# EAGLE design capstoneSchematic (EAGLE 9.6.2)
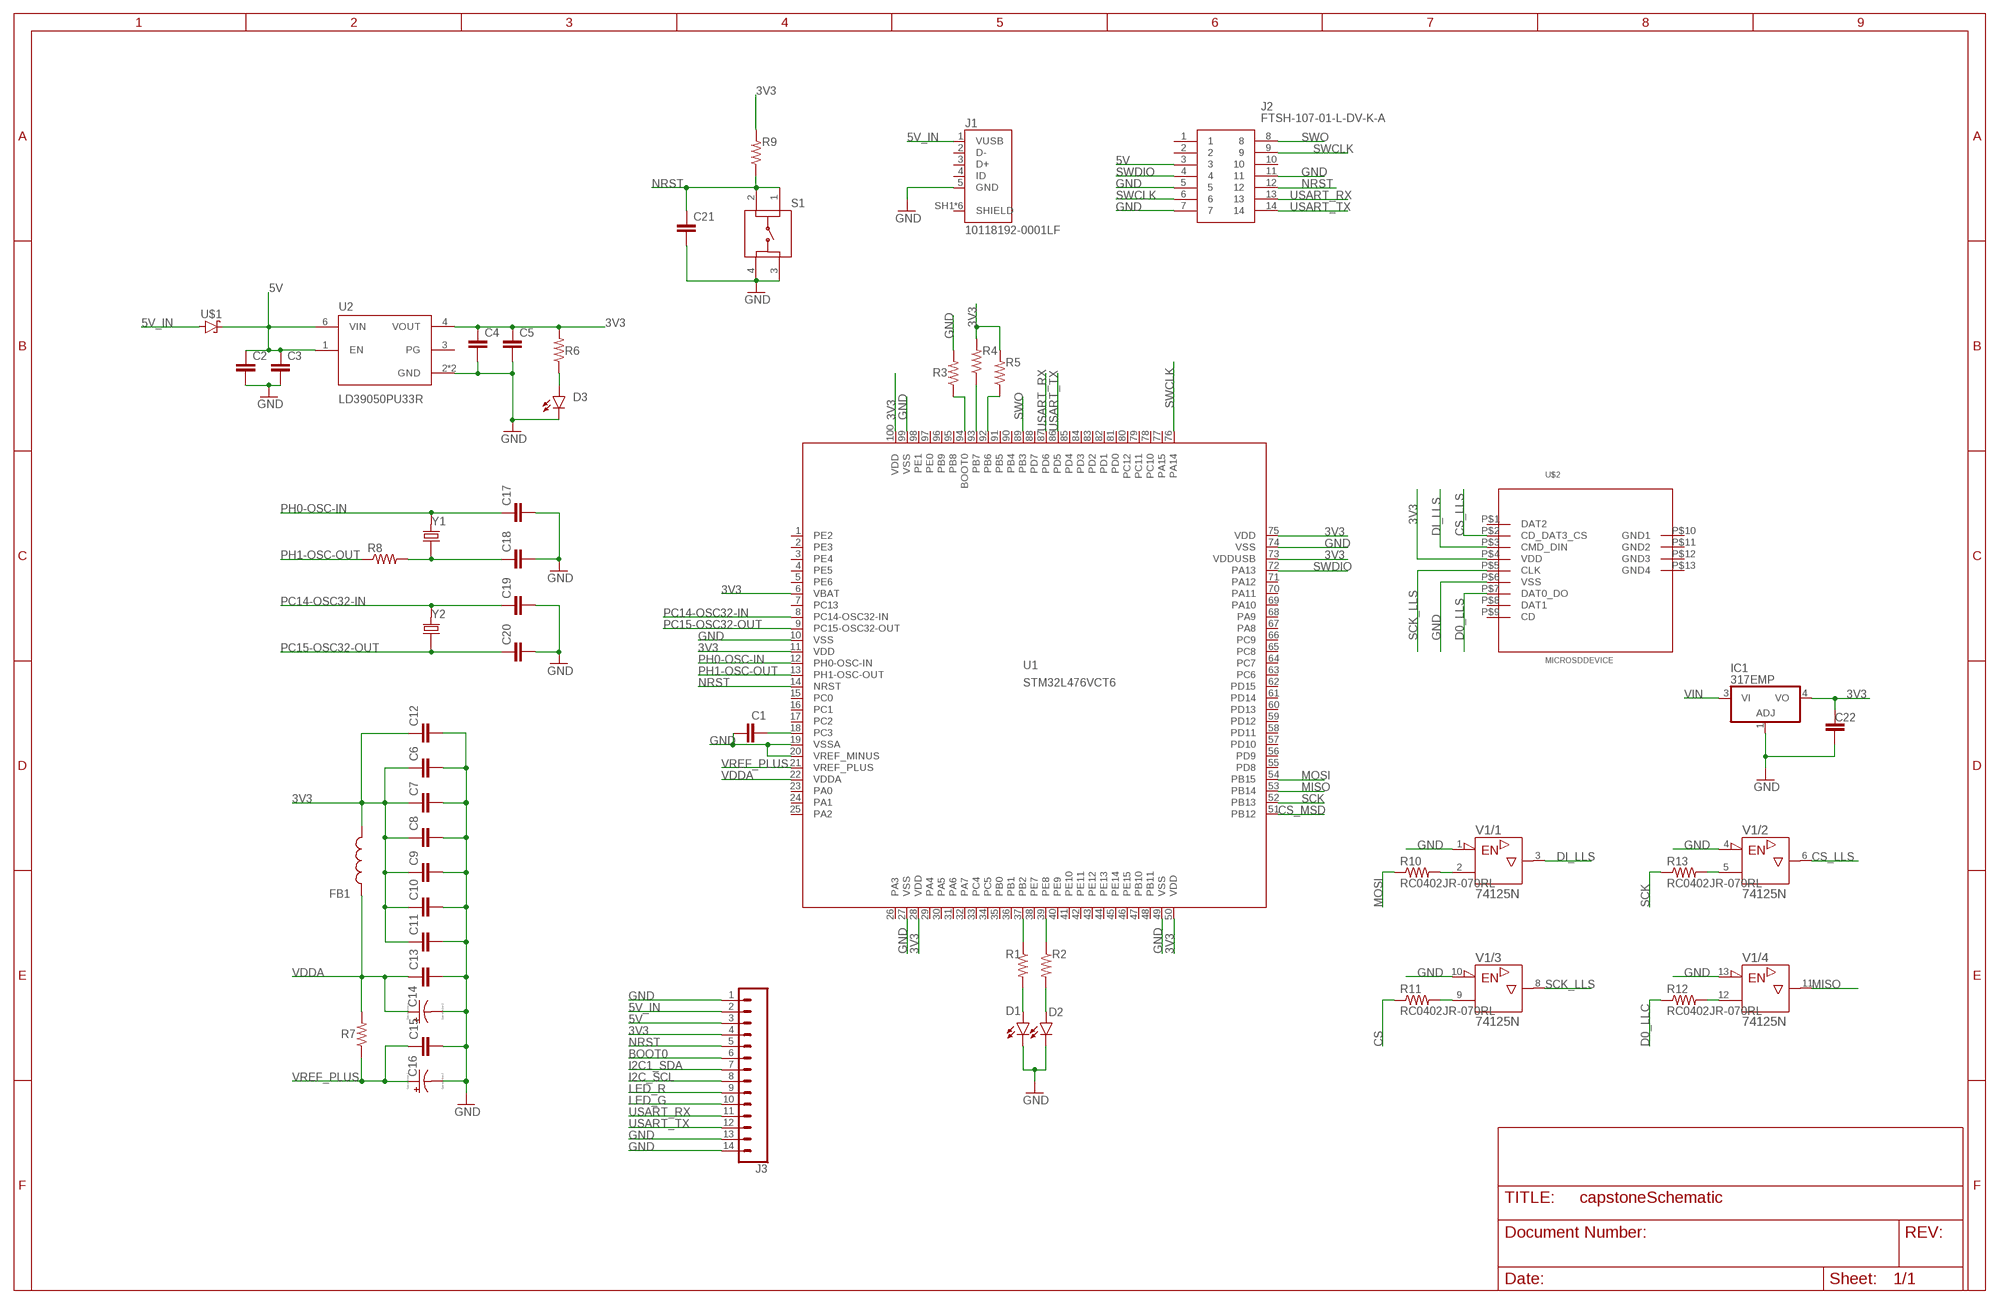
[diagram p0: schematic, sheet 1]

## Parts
C1  CC0603KRX5R7BB105  [CAPC1608X90]
C2  CC0603KRX5R7BB105  [CAPC1608X90]
C3  CC0402KRX7R7BB104  [CAPC1005X55N]
C4  CC0603KRX5R7BB105  [CAPC1608X90]
C5  CC0402KRX7R7BB104  [CAPC1005X55N]
C6  CC0402KRX7R7BB104  [CAPC1005X55N]
C7  CC0402KRX7R7BB104  [CAPC1005X55N]
C8  CC0402KRX7R7BB104  [CAPC1005X55N]
C9  CC0402KRX7R7BB104  [CAPC1005X55N]
C10  CC0402KRX7R7BB104  [CAPC1005X55N]
C11  CC0402KRX7R7BB104  [CAPC1005X55N]
C12  CC0603KRX5R7BB105  [CAPC1608X90]
C13  CC0402KRX7R7BB104  [CAPC1005X55N]
C14  TAJA105K016RNJ  [CAPPM3216X180N]
C15  CC0402KRX7R7BB104  [CAPC1005X55N]
C16  TAJA105K016RNJ  [CAPPM3216X180N]
C17  CC0402JRNPO9BN200  [CAPC1005X55N]
C18  CC0402JRNPO9BN200  [CAPC1005X55N]
C19  CC0402CRNPO9BN4R7  [CAPC1005X55N]
C20  CC0402CRNPO9BN4R7  [CAPC1005X55N]
C21  CC0402KRX7R7BB104  [CAPC1005X55N]
C22  C  (no package)
D1  SML-P12MTT86  [LED_SML-P11UTT86R]
D2  SML-P12MTT86  [LED_SML-P11UTT86R]
D3  SML-P12MTT86  [LED_SML-P11UTT86R]
FB1  BK1608HS601-T  [BEADC1608X95N]
IC1  317EMP  [SOT223]
J1  10118192-0001LF  [AMPHENOL_10118192-0001LF]
J2  FTSH-107-01-L-DV-K-A  [FTSH10701LDVKA]
J3  CONN_14  [1X14]
R1  RC0402FR-071KL  [RESC1005X40N]
R2  RC0402FR-071KL  [RESC1005X40N]
R3  RC0402FR-071KL  [RESC1005X40N]
R4  RC0402FR-071KL  [RESC1005X40N]
R5  RC0402FR-071KL  [RESC1005X40N]
R6  RC0402FR-071KL  [RESC1005X40N]
R7  RC0402FR-071KL  [RESC1005X40N]
R8  RC0402FR-072KL  [RESC1005X40N]
R9  RC0402FR-0710KL  [RESC1005X40N]
R10  RC0402JR-070RL  [RESC1005X40]
R11  RC0402JR-070RL  [RESC1005X40]
R12  RC0402JR-070RL  [RESC1005X40]
R13  RC0402JR-070RL  [RESC1005X40]
S1  LL3301FF065QJ  [LL3301FF065QJ]
U1  STM32L476VCT6  [LQFP100_14X14]
U2  LD39050PU33R  [SON95P300X300X100-7N]
U$1  STPS1L30A  [DIOM5226X223N]
U$2  MICROSDDEVICE  [MICROSD]
V1  74125N  [DIL14]
Y1  ABLS-8.000MHZ-B2-T  [XTAL_ABLS-8.000MHZ-B2-T]
Y2  ECS-.327-12.5-12QS-TR  [XTAL_ECS-.327-12.5-12QS-TR]

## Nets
3V3: C4.1 C5.1 C6.1 C7.1 C8.1 C9.1 C10.1 C11.1 C12.1 C22.1 FB1.2 IC1.4(VO) J3.4 R4.2 R5.2 R6.2 R9.2 U1.6(VBAT) U1.11(VDD) U1.28(VDD) U1.50(VDD) U1.73(VDDUSB) U1.75(VDD) U1.100(VDD) U2.4(VOUT) U$2.P$4(VDD)
5V: C2.1 C3.1 J2.3 J3.3 U2.1(EN) U2.6(VIN) U$1.1(C)
5V_IN: J1.1(VUSB) J3.2 U$1.2(A)
BOOT0: J3.6
CS: R11.1
CS_LLS: U$2.P$2(CD_DAT3_CS) V1.6(/2:Y)
CS_MSD: U1.51(PB12)
D0_LLC: R12.1
D0_LLS: U$2.P$7(DAT0_DO)
DI_LLS: U$2.P$3(CMD_DIN) V1.3(/1:Y)
GND: C1.1 C2.2 C3.2 C4.2 C5.2 C6.2 C7.2 C8.2 C9.2 C10.2 C11.2 C12.2 C13.2 C14.C(-) C15.2 C16.C(-) C17.2 C18.2 C19.2 C20.2 C21.2 C22.2 D1.C D2.C D3.C IC1.1(ADJ) J1.5(GND) J2.5 J2.7 J2.11 J3.1 J3.13 J3.14 R3.2 S1.3 S1.4 U1.10(VSS) U1.19(VSSA) U1.20(VREF_MINUS) U1.27(VSS) U1.49(VSS) U1.74(VSS) U1.99(VSS) U2.2(GND) U2.7(GND) U$2.P$6(VSS) V1.1(/1:!G) V1.4(/2:!G) V1.10(/3:!G) V1.13(/4:!G)
I2C1_SDA: J3.7
I2C_SCL: J3.8
LED_G: J3.10
LED_R: J3.9
MISO: U1.53(PB14) V1.11(/4:Y)
MOSI: R10.1 U1.54(PB15)
N$1: R2.1 U1.39(PE8)
N$2: R1.1 U1.37(PB2)
N$3: D1.A R1.2
N$4: D2.A R2.2
N$5: R3.1 U1.94(BOOT0)
N$6: R4.1 U1.93(PB7)
N$7: R5.1 U1.92(PB6)
N$8: D3.A R6.1
N$10: C1.2 U1.18(PC3)
N$12: C18.1 R8.2 Y1.1
N$13: R10.2 V1.2(/1:A)
N$15: R11.2 V1.9(/3:A)
N$17: R13.2 V1.5(/2:A)
N$21: R12.2 V1.12(/4:A)
NRST: C21.1 J2.12 J3.5 R9.1 S1.1 S1.2 U1.14(NRST)
PC14-OSC32-IN: C19.1 U1.8(PC14-OSC32-IN) Y2.2
PC15-OSC32-OUT: C20.1 U1.9(PC15-OSC32-OUT) Y2.1
PH0-OSC-IN: C17.1 U1.12(PH0-OSC-IN) Y1.2
PH1-OSC-OUT: R8.1 U1.13(PH1-OSC-OUT)
SCK: R13.1 U1.52(PB13)
SCK_LLS: U$2.P$5(CLK) V1.8(/3:Y)
SWCLK: J2.6 J2.9 U1.76(PA14)
SWDIO: J2.4 U1.72(PA13)
SWO: J2.8 U1.89(PB3)
USART_RX: J2.13 J3.11 U1.87(PD6)
USART_TX: J2.14 J3.12 U1.86(PD5)
VDDA: C13.1 C14.A(+) FB1.1 R7.2 U1.22(VDDA)
VIN: IC1.3(VI)
VREF_PLUS: C15.1 C16.A(+) R7.1 U1.21(VREF_PLUS)
Unconnected: J1.2(D-) J1.3(D+) J1.4(ID) J1.SH1(SHIELD) J1.SH2(SHIELD) J1.SH3(SHIELD) J1.SH4(SHIELD) J1.SH5(SHIELD) J1.SH6(SHIELD) J2.1 J2.2 J2.10 U1.1(PE2) U1.2(PE3) U1.3(PE4) U1.4(PE5) U1.5(PE6) U1.7(PC13) U1.15(PC0) U1.16(PC1) U1.17(PC2) U1.23(PA0) U1.24(PA1) U1.25(PA2) U1.26(PA3) U1.29(PA4) U1.30(PA5) U1.31(PA6) U1.32(PA7) U1.33(PC4) U1.34(PC5) U1.35(PB0) U1.36(PB1) U1.38(PE7) U1.40(PE9) U1.41(PE10) U1.42(PE11) U1.43(PE12) U1.44(PE13) U1.45(PE14) U1.46(PE15) U1.47(PB10) U1.48(PB11) U1.55(PD8) U1.56(PD9) U1.57(PD10) U1.58(PD11) U1.59(PD12) U1.60(PD13) U1.61(PD14) U1.62(PD15) U1.63(PC6) U1.64(PC7) U1.65(PC8) U1.66(PC9) U1.67(PA8) U1.68(PA9) U1.69(PA10) U1.70(PA11) U1.71(PA12) U1.77(PA15) U1.78(PC10) U1.79(PC11) U1.80(PC12) U1.81(PD0) U1.82(PD1) U1.83(PD2) U1.84(PD3) U1.85(PD4) U1.88(PD7) U1.90(PB4) U1.91(PB5) U1.95(PB8) U1.96(PB9) U1.97(PE0) U1.98(PE1) U2.3(PG) U$2.P$1(DAT2) U$2.P$8(DAT1) U$2.P$9(CD) U$2.P$10(GND1) U$2.P$11(GND2) U$2.P$12(GND3) U$2.P$13(GND4)

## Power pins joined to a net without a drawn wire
+UB: V1.14(/+UB:+UB)
-UB: V1.7(/-UB:-UB)

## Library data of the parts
C1 C2 C4 C12 = ce-capstone:CC0603KRX5R7BB105: CAPACITOR CERAMIC, 1µF, 10V, X5R, 0603; Dielectric Characteristic:X5R; Capacitance:1µF; Capacitance Tolerance:± 10%; Voltage Rating:16V; Temperature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; DESCRIPTION: 1µF ±10% 16V Ceramic Capacitor X5R 0603 _1608 Metric_; DIGI-KEY_PART_NUMBER: 311-1444-1-ND; DIGI-KEY_PURCHASE_URL: https://www.digikey.com/product-detail/en/yageo/CC0603KRX5R7BB105/311-1444-1-ND/2833750?utm_source=snapeda&utm_medium=aggregator&utm_campaign=symbol; MF: Yageo; MP: CC0603KRX5R7BB105; PACKAGE: 0603 Yageo
C3 C5-C11 C13 C15 C21 = ce-capstone:CC0402KRX7R7BB104: .1UF 16V 10% 0402; DESCRIPTION: 0.1µF ±10% 16V Ceramic Capacitor X7R 0402 _1005 Metric_; DIGI-KEY_PART_NUMBER: 311-1338-1-ND; DIGI-KEY_PURCHASE_URL: https://www.digikey.com/product-detail/en/yageo/CC0402KRX7R7BB104/311-1338-1-ND/2103122?utm_source=snapeda&utm_medium=aggregator&utm_campaign=symbol; MF: Yageo; MP: CC0402KRX7R7BB104; PACKAGE: 0402 Yageo
C14 C16 = ce-capstone:TAJA105K016RNJ: Capacitor tantalum TAJ 1206 1uF 16V AVX 1uF SMD Solid MnO2 Tantalum Electrolytic Capacitor, 16 V dc +/-10%, TAJ Series; ALLIED_NUMBER: 70474975; ALLIED_PRICE-STOCK: https://www.alliedelec.com/avx-taja105k016r/70474975/; DESCRIPTION: Capacitor tantalum TAJ 1206 1uF 16V AVX 1uF SMD Solid MnO2 Tantalum Electrolytic Capacitor, 16 V dc +/-10%, TAJ Series; HEIGHT: 1.8mm; MANUFACTURER_NAME: AVX; MANUFACTURER_PART_NUMBER: TAJA105K016RNJ; MOUSER_PART_NUMBER: 581-TAJA105K016RNJ; MOUSER_PRICE-STOCK: https://www.mouser.com/Search/Refine.aspx?Keyword=581-TAJA105K016R; RS_PART_NUMBER: 6992804P; RS_PRICE-STOCK: http://uk.rs-online.com/web/p/products/6992804P
C17 C18 = ce-capstone:CC0402JRNPO9BN200: CAPACITOR CERAMIC 20PF 50V, C0G, 0402; Dielectric Characteristic:C0G / NP0; Capacitance:20pF; Capacitance Tolerance:± 5%; Voltage Rating:50V; Capacitor Case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; DESCRIPTION: 20pF ±5% 50V Ceramic Capacitor C0G, NP0 0402 _1005 Metric_; DIGI-KEY_PART_NUMBER: 311-1417-1-ND; DIGI-KEY_PURCHASE_URL: https://www.digikey.com/product-detail/en/yageo/CC0402JRNPO9BN200/311-1417-1-ND/2833723?utm_source=snapeda&utm_medium=aggregator&utm_campaign=symbol; MF: Yageo; MP: CC0402JRNPO9BN200; PACKAGE: 0402 Yageo
C19 C20 = ce-capstone:CC0402CRNPO9BN4R7: 0402 4.7 pF 50 V ±0.25 pF Tolerance NP0 SMT Multilayer Ceramic Capacitor; DESCRIPTION: 4.7pF ±0.25pF 50V Ceramic Capacitor C0G, NP0 0402 _1005 Metric_; DIGI-KEY_PART_NUMBER: 311-1367-1-ND; DIGI-KEY_PURCHASE_URL: https://www.digikey.com/product-detail/en/yageo/CC0402CRNPO9BN4R7/311-1367-1-ND/2103151?utm_source=snapeda&utm_medium=aggregator&utm_campaign=symbol; MF: Yageo; MP: CC0402CRNPO9BN4R7; PACKAGE: 0402 Yageo
C22 = ngspice-simulation:C: CAPACITOR
D1-D3 = ce-capstone:SML-P12MTT86: SML-P1 Series Red 0402 Clear 60 mcd 2 V Surface Mount PICOLED LED; AVAILABILITY: Unavailable; DESCRIPTION: Green 572nm LED Indication - Discrete 2V 0402 _1006 Metric_; MF: Rohm; MP: SML-P12MTT86; PACKAGE: 0402 Rohm; PRICE: None
FB1 = ce-capstone:BK1608HS601-T: Ferrite Chip Bead(Lead Free); DESCRIPTION: Ferrite Chip Bead(Lead Free); HEIGHT: 0.95mm; MANUFACTURER_NAME: Taiyo Yuden; MANUFACTURER_PART_NUMBER: BK1608HS601-T
IC1 = linear:*317: Positive VOLTAGE REGULATOR
J1 = ce-capstone:10118192-0001LF: Single Port 5 Contact Horizontal Right Angle Shielded Micro B USB 2.0 Connector; AVAILABILITY: Unavailable; DESCRIPTION: USB - micro B USB 2.0 Receptacle Connector 5 Position Surface Mount, Right Angle; MF: Amphenol ICC; MP: 10118192-0001LF; PACKAGE: None; PRICE: None
J2 = ce-capstone:FTSH-107-01-L-DV-K-A: Headers & Wire Housings .050" Micro Terminal Strip Source: Datasheet; DESCRIPTION: Headers & Wire Housings .050" Micro Terminal Strip; HEIGHT: 5.97mm; MANUFACTURER_NAME: SAMTEC; MANUFACTURER_PART_NUMBER: FTSH-107-01-L-DV-K-A; MOUSER_PART_NUMBER: 200-FTSH10701LDVKA; MOUSER_PRICE-STOCK: https://www.mouser.com/Search/Refine.aspx?Keyword=200-FTSH10701LDVKA
J3 = SparkFun-Connectors:CONN_14: Multi connection point. Often used as Generic Header-pin footprint for 0.1 inch spaced/style header connections On any of the 0.1 inch spaced packages, you can populate with these: Break Away Headers - Straight (PRT-00116) Break Away Male Headers - Right Angle (PRT-00553) Female Headers (PRT-00115)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
R1-R7 = ce-capstone:RC0402FR-071KL: RES SMD 1k OHM 1% 1/16W 0402; DESCRIPTION: 510 Ohms ±1% 0.063W, 1/16W Chip Resistor 0402 _1005 Metric_ Moisture Resistant Thick Film; DIGI-KEY_PART_NUMBER: 311-510LRCT-ND; DIGI-KEY_PURCHASE_URL: https://www.digikey.com/product-detail/en/yageo/RC0402FR-07510RL/311-510LRCT-ND/729579?utm_source=snapeda&utm_medium=aggregator&utm_campaign=symbol; MF: Yageo; MP: RC0402FR-07510RL; PACKAGE: 1005 Panasonic Electronic Components
R8 = ce-capstone:RC0402FR-072KL: RES SMD 2k OHM 1% 1/16W 0402; DESCRIPTION: 510 Ohms ±1% 0.063W, 1/16W Chip Resistor 0402 _1005 Metric_ Moisture Resistant Thick Film; DIGI-KEY_PART_NUMBER: 311-510LRCT-ND; DIGI-KEY_PURCHASE_URL: https://www.digikey.com/product-detail/en/yageo/RC0402FR-07510RL/311-510LRCT-ND/729579?utm_source=snapeda&utm_medium=aggregator&utm_campaign=symbol; MF: Yageo; MP: RC0402FR-07510RL; PACKAGE: 1005 Panasonic Electronic Components
R9 = ce-capstone:RC0402FR-0710KL: RES SMD 10k OHM 1% 1/16W 0402; DESCRIPTION: 510 Ohms ±1% 0.063W, 1/16W Chip Resistor 0402 _1005 Metric_ Moisture Resistant Thick Film; DIGI-KEY_PART_NUMBER: 311-510LRCT-ND; DIGI-KEY_PURCHASE_URL: https://www.digikey.com/product-detail/en/yageo/RC0402FR-07510RL/311-510LRCT-ND/729579?utm_source=snapeda&utm_medium=aggregator&utm_campaign=symbol; MF: Yageo; MP: RC0402FR-07510RL; PACKAGE: 1005 Panasonic Electronic Components
R10-R13 = ce-capstone:RC0402JR-070RL: RC Series 0402 62.5 mW 0 Ohms 5% ±200 ppm/°C SMT Thick Film Chip Resistor; AVAILABILITY: Unavailable; DESCRIPTION: 0 Ohms Jumper 0.063W, 1/16W Chip Resistor 0402 _1005 Metric_ Moisture Resistant Thick Film; MF: Yageo; MP: RC0402JR-070RL; PACKAGE: 0402 Yageo; PRICE: None
S1 = ce-capstone:LL3301FF065QJ: Pushbutton Switches 50mA 12VDC F065 7.0mm J-Lead Source: Datasheet; DESCRIPTION: Pushbutton Switches 50mA 12VDC F065 7.0mm J-Lead; HEIGHT: 7.3mm; MANUFACTURER_NAME: E-Switch; MANUFACTURER_PART_NUMBER: LL3301FF065QJ; MOUSER_PART_NUMBER: 612-LL3301FF065QJ; MOUSER_PRICE-STOCK: https://www.mouser.com/Search/Refine.aspx?Keyword=612-LL3301FF065QJ
U1 = ce-capstone:STM32L476V*: STM32L476VX LQFP100 Datasheet STM32L476XX; FARNELL: 2518171; FLASH: 256kB; SRAM: 128kB
U2 = ce-capstone:LD39050PU33R: LD39050 Series 500 mA 3.3 V Fixed Low Noise LDO Voltage Regulator - DFN-6; AVAILABILITY: Unavailable; DESCRIPTION: Linear Voltage Regulator IC 1 Output 500mA 6-DFN _3x3_; MF: STMicroelectronics; MP: LD39050PU33R; PACKAGE: DFN-6 STMicroelectronics; PRICE: None
U$1 = ce-capstone:STPS1L30A
U$2 = MicroSDFootprint:MICROSDDEVICE
V1 = 74ttl-din:74*125: Quad bus BUFFER, 3-state
Y1 = ce-capstone:ABLS-8.000MHZ-B2-T: Crystal 8MHz Â±20ppm (Tol) Â±50ppm (Stability) 18pF FUND 80Ohm 2-Pin HC-49/US SMD T/R; AVAILABILITY: Unavailable; DESCRIPTION: 8MHz ±20ppm Crystal 18pF 80 Ohms HC-49/US; MF: Abracon LLC; MP: ABLS-8.000MHZ-B2; PACKAGE: HC-49/US Abracon LLC; PRICE: None
Y2 = ce-capstone:ECS-.327-12.5-12QS-TR: SMD CRYSTAL 32.768 KHz; AVAILABILITY: Unavailable; DESCRIPTION: 32.768kHz ±20ppm Crystal 12.5pF 90 kOhms 2-SMD, No Lead; MF: ECS Inc.; MP: ECS-.327-12.5-12QS-TR; PACKAGE: SMD-2 ECS International; PRICE: None

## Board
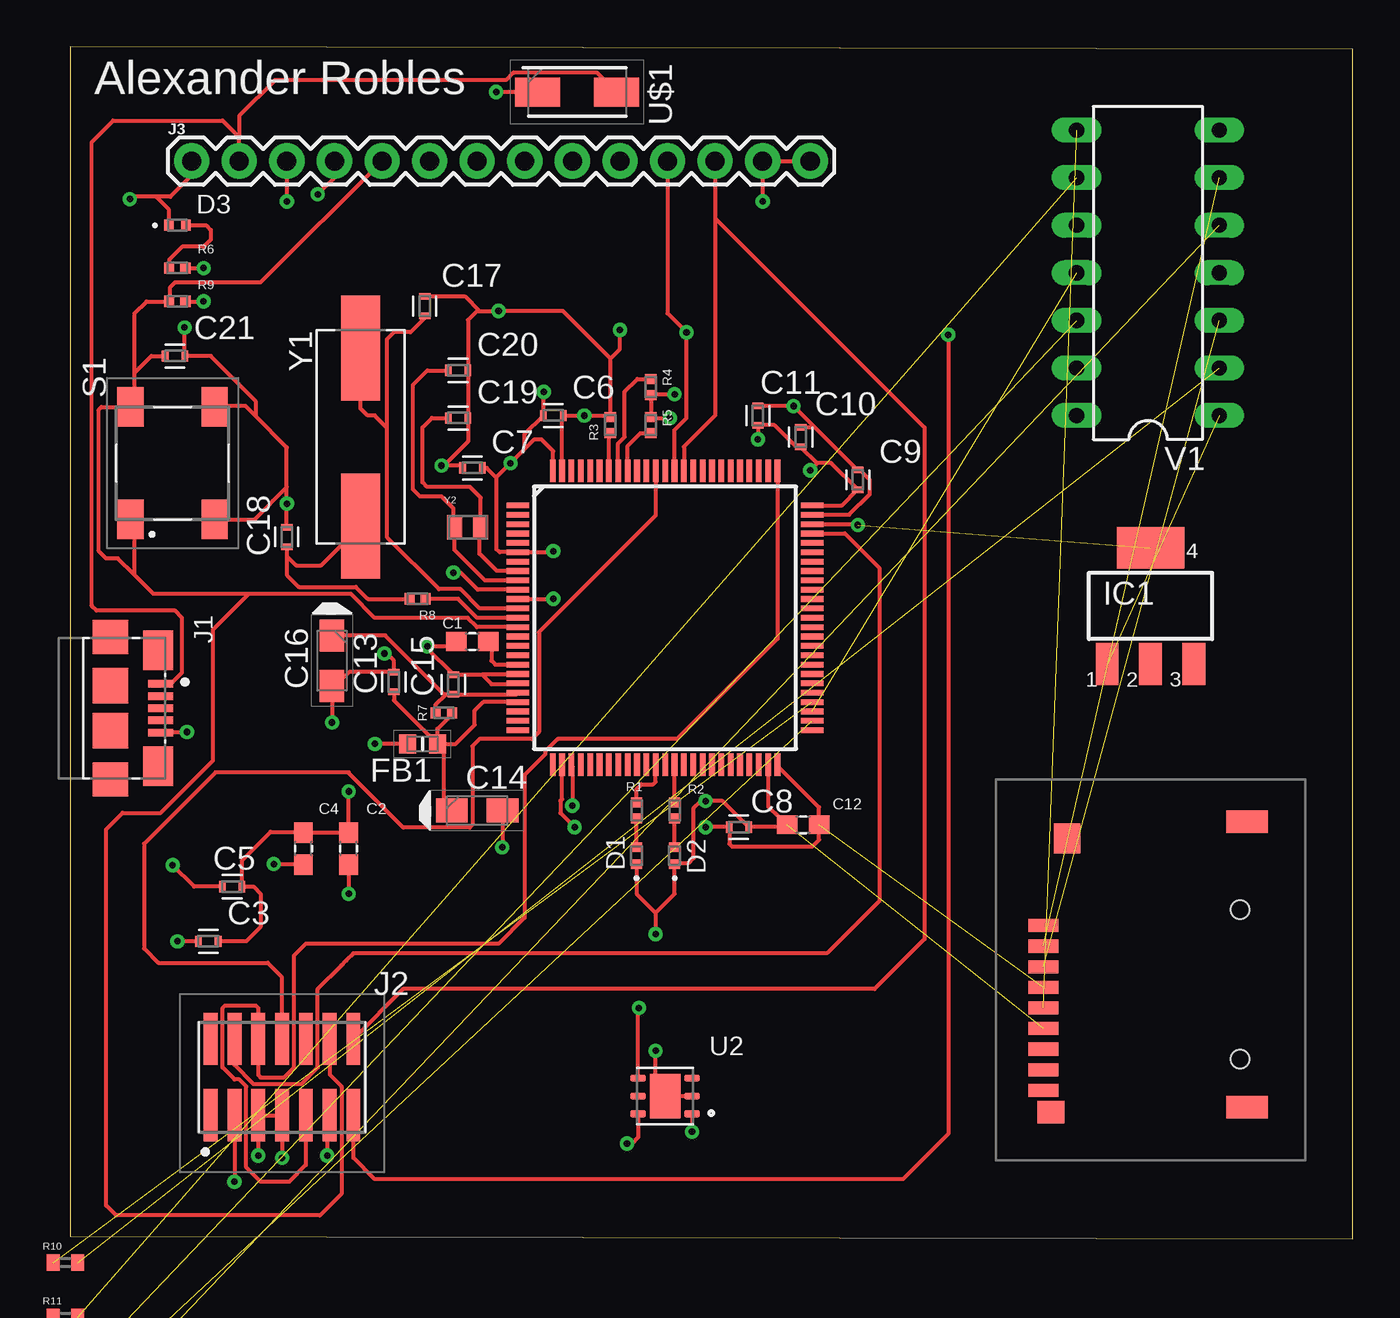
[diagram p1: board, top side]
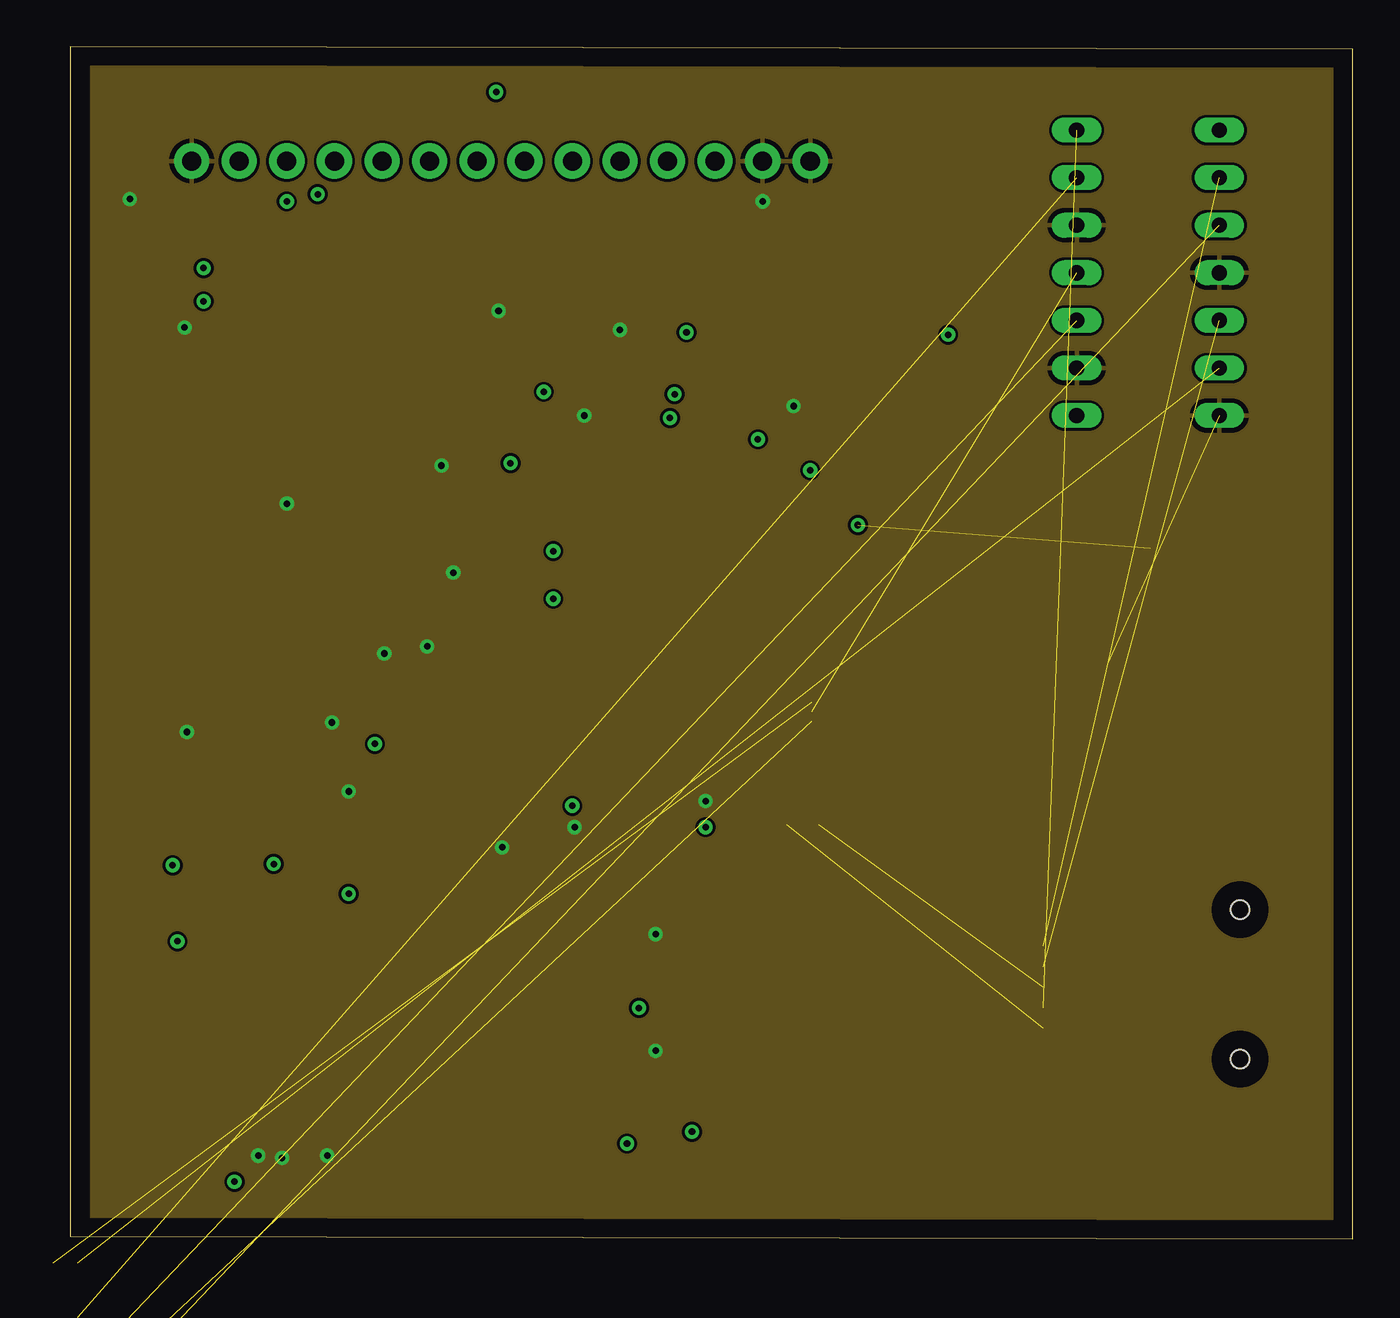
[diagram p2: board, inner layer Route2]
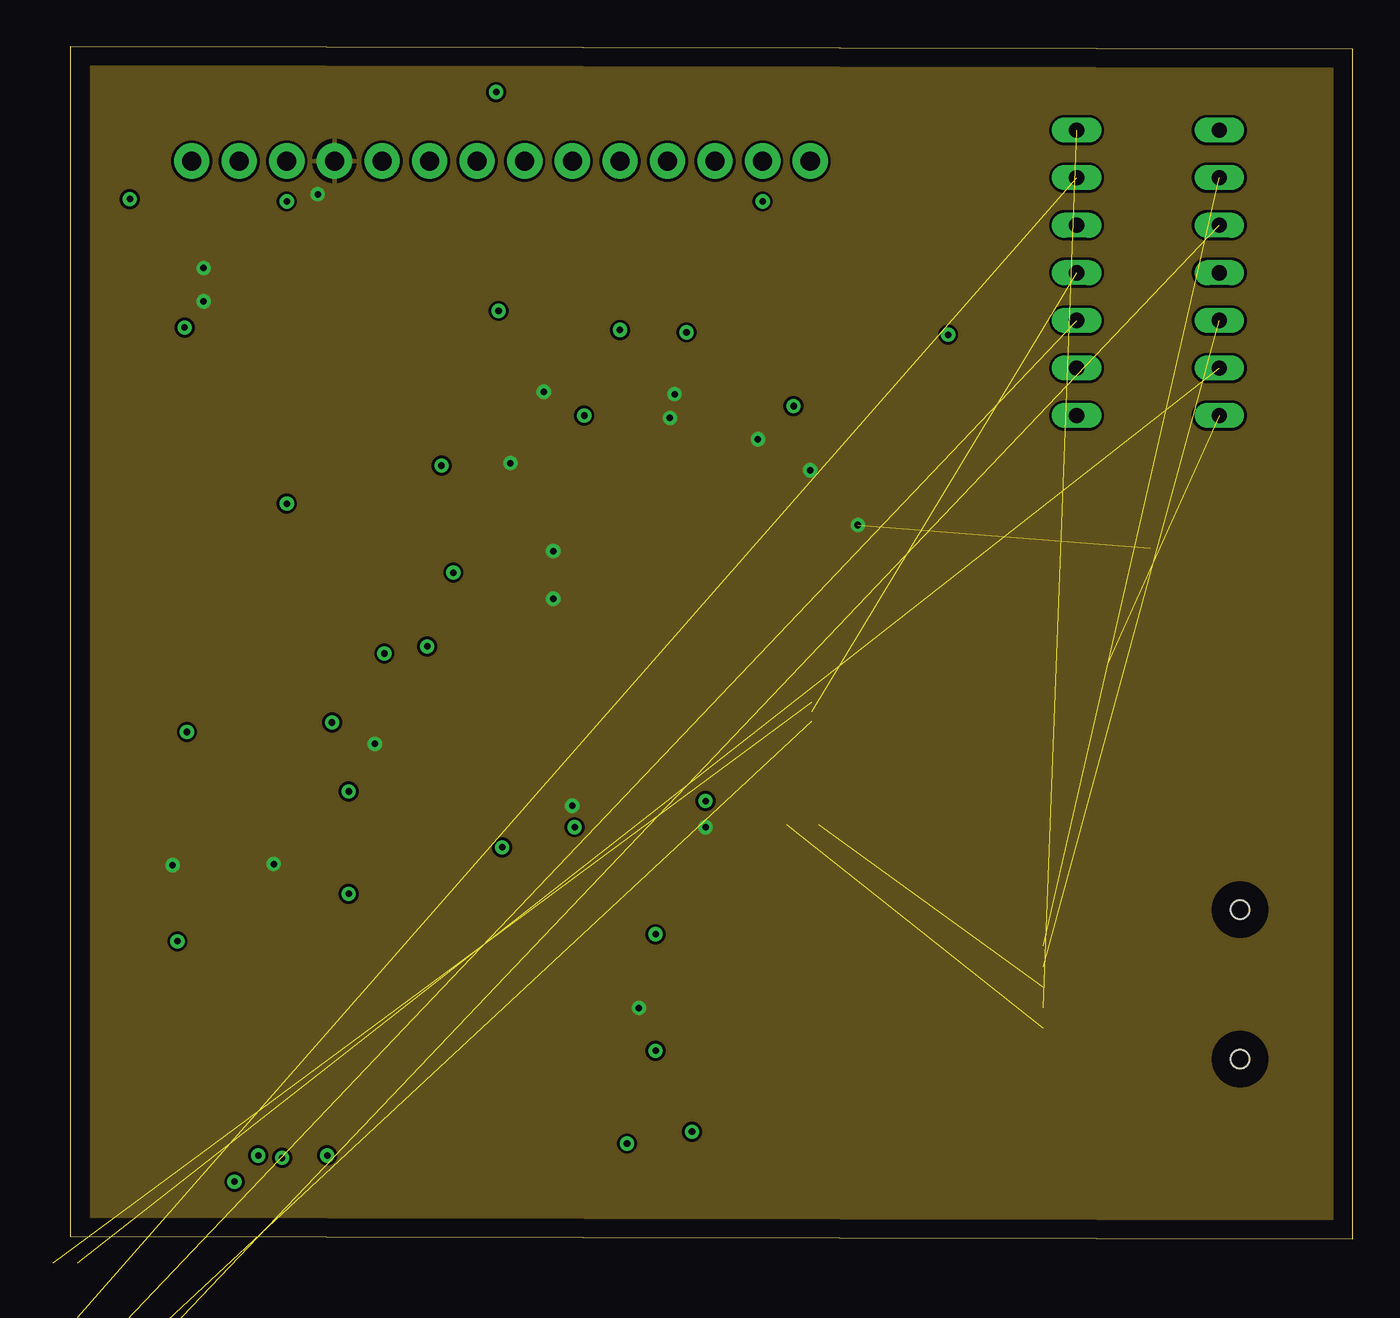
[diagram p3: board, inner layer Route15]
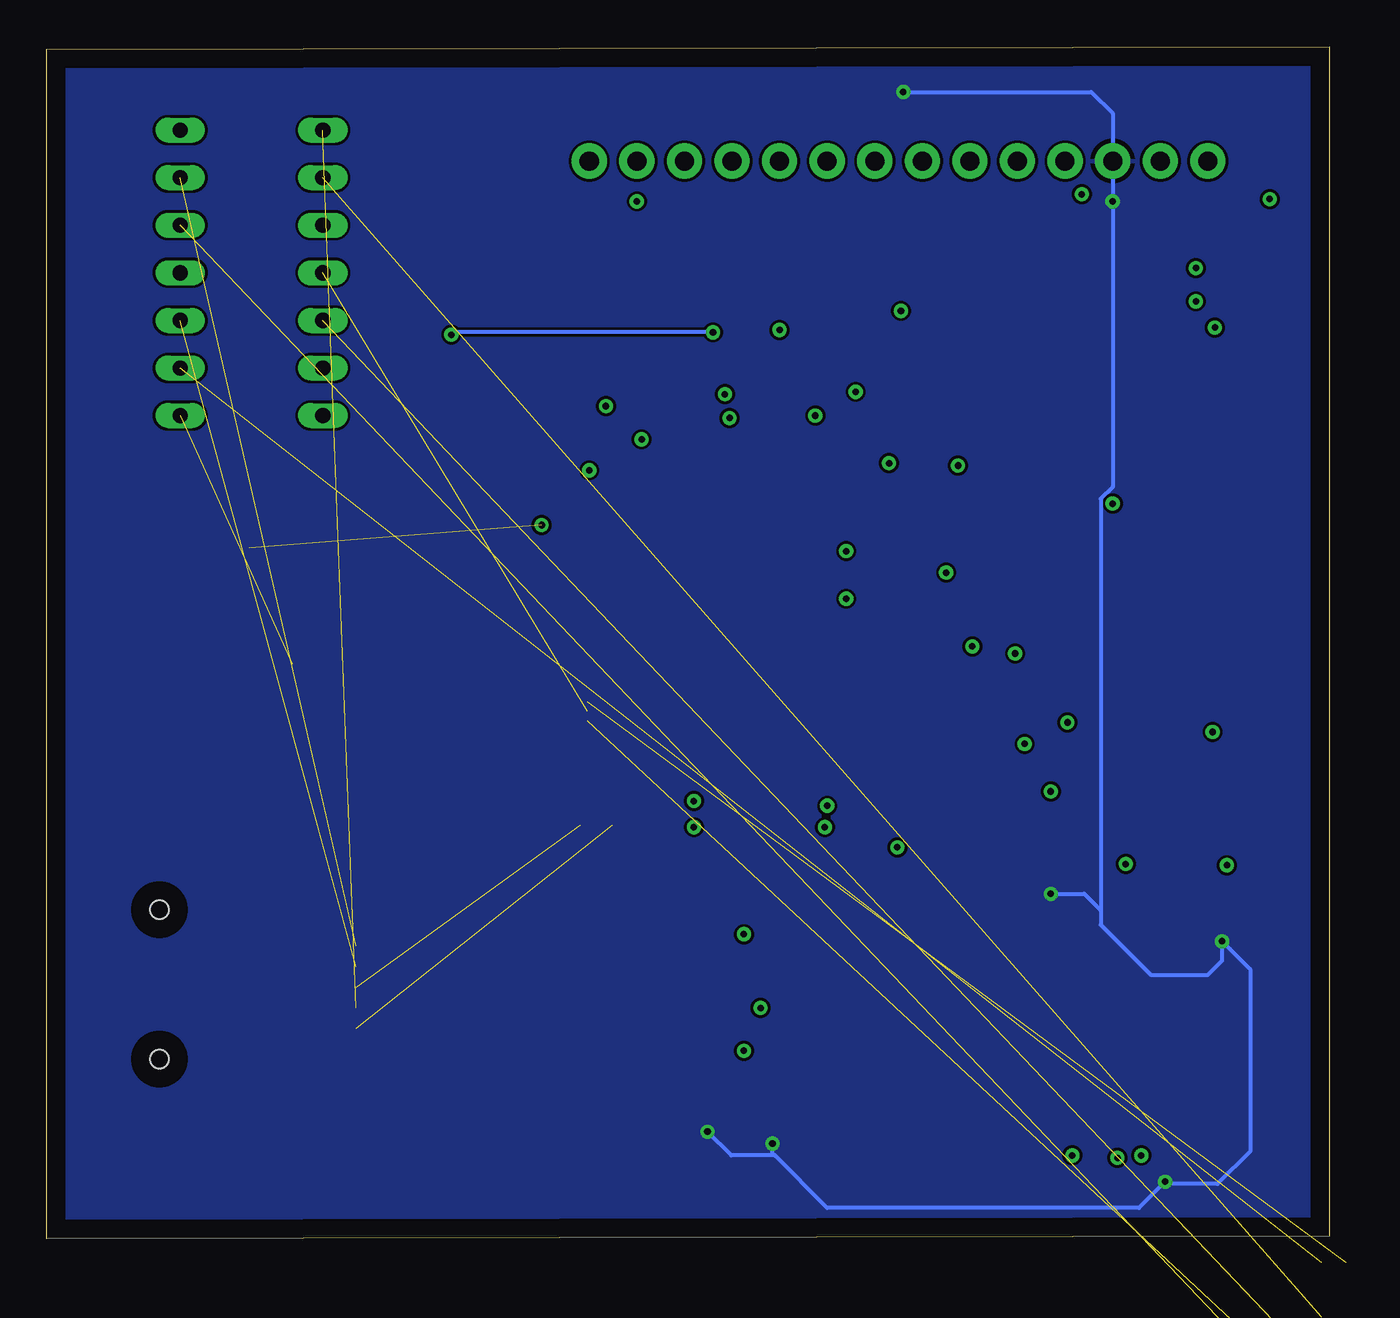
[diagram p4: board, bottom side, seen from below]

Size 68.45 x 63.63 mm. Coordinates in mm from the lower left corner, seen from the top.
Outline: 0,0.13 68.45,0 68.45,63.5 0,63.63 0,0.13
Copper layers (1+2*15+16): Top 0.035mm / dielectric 1.5mm / Route2 0.035mm / dielectric 0.15mm / Route15 0.035mm / dielectric 0.2mm / Bottom 0.035mm
Design rules "default *": minimum track width 8mil, minimum drill 0.35mm, track to track 6mil, track to pad 6mil, pad to pad 6mil, via to via 6mil, smd to smd 6mil, copper to edge 40mil, drill to drill 6mil, minimum pad ring 10mil, minimum via ring 8mil, stop-mask expansion 4mil, vias tented up to drill 0mil, thermal gap 10mil

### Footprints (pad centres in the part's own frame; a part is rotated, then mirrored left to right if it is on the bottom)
CAPC1608X90 = smd 1.1 x 1: 1 -0.85,0; 2 0.85,0
CAPC1005X55N = smd 0.35 x 0.6: 1 -0.525,0; 2 0.525,0
CAPPM3216X180N = smd 1.7 x 1.3: A -1.35,0; C 1.35,0
LED_SML-P11UTT86R = smd 0.5 x 0.6: A 0.45,0; C -0.45,0
BEADC1608X95N = smd 0.9 x 1: 1 -0.8,0; 2 0.8,0
SOT223 = smd 1.219 x 2.235: 1 -2.311,-3.099; 2 0,-3.099; 3 2.311,-3.099 | smd 3.6 x 2.2: 4 0,3.099
AMPHENOL_10118192-0001LF = smd 0.4 x 1.35: 1 -1.3,0; 2 -0.65,0; 3 0,0; 4 0.65,0; 5 1.3,0 | smd 2.1 x 1.6: SH1 -3.1,-0.125; SH2 3.1,-0.125 | smd 1.8 x 1.9: SH3 -3.8,-2.675; SH6 3.8,-2.675 | smd 1.9 x 1.9: SH4 -1.2,-2.675; SH5 1.2,-2.675
FTSH10701LDVKA = smd 0.74 x 2.79: 1 -3.81,-2.035; 2 -3.81,2.035; 3 -2.54,-2.035; 4 -2.54,2.035; 5 -1.27,-2.035; 6 -1.27,2.035; 7 0,-2.035; 8 0,2.035; 9 1.27,-2.035; 10 1.27,2.035; 11 2.54,-2.035; 12 2.54,2.035; 13 3.81,-2.035; 14 3.81,2.035
1X14 = drill 1.016 pad 1.88: 1 0,0; 2 2.54,0; 3 5.08,0; 4 7.62,0; 5 10.16,0; 6 12.7,0; 7 15.24,0; 8 17.78,0; 9 20.32,0; 10 22.86,0; 11 25.4,0; 12 27.94,0; 13 30.48,0; 14 33.02,0
RESC1005X40N = smd 0.54 x 0.6: 1 -0.432,0; 2 0.432,0
RESC1005X40 = smd 0.7 x 0.9: 1 -0.65,0; 2 0.65,0
LL3301FF065QJ = smd 2.1 x 1.4: 1 -3,2.25; 2 3,2.25; 3 -3,-2.25; 4 3,-2.25
LQFP100_14X14 = smd 1.2 x 0.3: 1 -7.85,6; 2 -7.85,5.5; 3 -7.85,5; 4 -7.85,4.5; 5 -7.85,4; 6 -7.85,3.5; 7 -7.85,3; 8 -7.85,2.5; 9 -7.85,2; 10 -7.85,1.5; 11 -7.85,1; 12 -7.85,0.5; 13 -7.85,0; 14 -7.85,-0.5; 15 -7.85,-1; 16 -7.85,-1.5; 17 -7.85,-2; 18 -7.85,-2.5; 19 -7.85,-3; 20 -7.85,-3.5; 21 -7.85,-4; 22 -7.85,-4.5; 23 -7.85,-5; 24 -7.85,-5.5; 25 -7.85,-6; 51 7.85,-6; 52 7.85,-5.5; 53 7.85,-5; 54 7.85,-4.5; 55 7.85,-4; 56 7.85,-3.5; 57 7.85,-3; 58 7.85,-2.5; 59 7.85,-2; 60 7.85,-1.5; 61 7.85,-1; 62 7.85,-0.5; 63 7.85,0; 64 7.85,0.5; 65 7.85,1; 66 7.85,1.5; 67 7.85,2; 68 7.85,2.5; 69 7.85,3; 70 7.85,3.5; 71 7.85,4; 72 7.85,4.5; 73 7.85,5; 74 7.85,5.5; 75 7.85,6 | smd 0.3 x 1.2: 26 -6,-7.85; 27 -5.5,-7.85; 28 -5,-7.85; 29 -4.5,-7.85; 30 -4,-7.85; 31 -3.5,-7.85; 32 -3,-7.85; 33 -2.5,-7.85; 34 -2,-7.85; 35 -1.5,-7.85; 36 -1,-7.85; 37 -0.5,-7.85; 38 0,-7.85; 39 0.5,-7.85; 40 1,-7.85; 41 1.5,-7.85; 42 2,-7.85; 43 2.5,-7.85; 44 3,-7.85; 45 3.5,-7.85; 46 4,-7.85; 47 4.5,-7.85; 48 5,-7.85; 49 5.5,-7.85; 50 6,-7.85; 76 6,7.85; 77 5.5,7.85; 78 5,7.85; 79 4.5,7.85; 80 4,7.85; 81 3.5,7.85; 82 3,7.85; 83 2.5,7.85; 84 2,7.85; 85 1.5,7.85; 86 1,7.85; 87 0.5,7.85; 88 0,7.85; 89 -0.5,7.85; 90 -1,7.85; 91 -1.5,7.85; 92 -2,7.85; 93 -2.5,7.85; 94 -3,7.85; 95 -3.5,7.85; 96 -4,7.85; 97 -4.5,7.85; 98 -5,7.85; 99 -5.5,7.85; 100 -6,7.85
SON95P300X300X100-7N = smd 0.84 x 0.4: 1 -1.435,0.95; 2 -1.435,0; 3 -1.435,-0.95; 4 1.435,-0.95; 5 1.435,0; 6 1.435,0.95 | smd 1.625 x 2.365: 7 0,0
DIOM5226X223N = smd 2.4 x 1.55: 1 -2.1,0; 2 2.1,0
MICROSD = smd 1.6 x 0.7: P$1 -3.81,1.1; P$2 -3.81,0; P$3 -3.81,-1.1; P$4 -3.81,-2.2; P$5 -3.81,-3.3; P$6 -3.81,-4.4; P$7 -3.81,-5.5; P$8 -3.81,-6.6; P$9 -3.81,-7.7 | smd 1.45 x 1.2: P$10 -3.41,-8.85 | smd 1.4 x 1.6: P$11 -2.54,5.75 | smd 2.2 x 1.2: P$12 7.06,6.65; P$13 7.06,-8.59 | hole 1: 6.69,1.95; 6.69,-6.03
DIL14 = drill 0.813 long: 1 -7.62,-3.81; 2 -5.08,-3.81; 3 -2.54,-3.81; 4 0,-3.81; 5 2.54,-3.81; 6 5.08,-3.81; 7 7.62,-3.81; 8 7.62,3.81; 9 5.08,3.81; 10 2.54,3.81; 11 0,3.81; 12 -2.54,3.81; 13 -5.08,3.81; 14 -7.62,3.81
XTAL_ABLS-8.000MHZ-B2-T = smd 5.6 x 2.1: 1 -4.75,0; 2 4.75,0
XTAL_ECS-.327-12.5-12QS-TR = smd 0.8 x 1.3: 1 -0.7,0; 2 0.7,0

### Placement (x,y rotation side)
C1  21.46,31.88 0 top
C2  14.86,20.83 90 top
C3  7.37,15.88 0 top
C4  12.45,20.83 90 top
C5  8.64,18.8 0 top
C6  25.78,43.94 0 top
C7  21.46,41.15 180 top
C8  35.69,21.97 0 top
C9  42.04,40.51 90 top
C10  38.99,42.8 90 top
C11  36.7,43.94 90 top
C12  39.12,22.1 180 top
C13  17.27,29.72 90 top
C14  21.72,22.86 0 top
C15  20.45,29.59 90 top
C16  13.97,30.86 270 top
C17  18.92,49.78 90 top
C18  11.56,37.47 90 top
C19  20.7,43.82 0 top
C20  20.7,46.36 0 top
C21  5.59,47.12 0 top
D1  30.23,20.45 90 top
D2  32.26,20.45 90 top
D3  5.71,54.1 0 top
FB1  18.8,26.42 180 top
IC1  57.66,33.78 0 top
J1  4.83,28.32 270 top
J2  11.3,8.64 0 top
J3  6.48,57.53 0 top
R1  30.23,22.86 270 top
R2  32.26,22.86 270 top
R3  28.83,43.43 90 top
R4  30.99,45.47 270 top
R5  30.99,43.43 90 top
R6  5.71,51.82 0 top
R7  19.94,28.07 0 top
R8  18.54,34.16 180 top
R9  5.71,50.04 0 top
R10  -0.25,-1.27 0 top
R11  not placed on the board
R12  not placed on the board
R13  not placed on the board
S1  5.46,41.4 90 top
U1  31.75,33.15 0 top
U2  31.75,7.62 180 top
U$1  27.05,61.21 0 top
U$2  55.75,15.62 0 top
V1  57.53,51.56 90 top
Y1  15.49,42.8 90 top
Y2  21.21,37.97 0 top

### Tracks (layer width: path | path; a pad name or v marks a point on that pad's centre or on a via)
3V3  (via drill 0.35)  (2 unrouted)
  Top 0.203: 22.73,40.64 22.73,36.83 22.92,36.65 U1.6 25.73,36.65 v25.78,36.7 | 22.73,40.64 v23.5,41.4 24.26,42.16 | 24.26,42.16 24.26,42.94 C6.1 25.26,45.2 v25.27,45.21 | U1.50 37.75,25.24 39.97,23.03 C12.1 39.97,21.3 39.62,20.95 35.31,20.95 35.18,21.08 35.18,21.95 C8.1 v33.91,21.97 | U1.75 41.18,39.15 42.02,39.99 C9.1 40.64,41.39 40.64,41.4 39.88,41.4 | 39.88,41.4 39.86,41.4 C10.1 38.75,42.27 37.59,43.43 36.72,43.43 C11.1 v36.7,42.67 | 39.88,41.4 v39.5,41.02 | FB1.2 v16.26,26.42 | v32.26,45.09 31.04,45.09 R4.2 R5.2 31.04,43.82 v32,43.82 | C7.1 22.23,41.15 22.73,40.64 | U1.100 25.78,41.03 25.78,42.04 25.15,42.67 24.77,42.67 24.26,42.16 | U1.28 26.8,25.25 v26.8,23.11 | U2.4 30.32,12.28 v30.35,12.32 | C5.1 6.6,18.8 v5.46,19.94 | J3.4 14.1,56.64 v13.21,55.75 | R9.2 v7.11,50.04 | R6.2 v7.11,51.82 | U1.73 41.99,38.15 v42.04,38.1 | U1.11 25.77,34.15 v25.78,34.16 | C4.1 10.88,19.98 v10.86,20
  pour Route15: 0.76,63.12 68.07,63.12 68.07,0.38 0.76,0.38
5V  (via drill 0.35)
  Top 0.203: U2.1 v33.19,5.71 | U2.6 30.32,5.42 29.97,5.08 v29.72,5.08 | J2.3 v8.76,3.05 | J3.3 v11.56,55.37 | C2.1 v14.86,18.41 | C3.1 v5.71,15.88 | U$1.1 v22.73,61.21
  Bottom 0.203: 12.19,17.53 12.19,39.51 11.56,40.14 v11.56,55.37 11.56,60.07 12.7,61.21 v22.73,61.21 | 12.19,17.53 12.19,16.76 9.53,14.1 6.48,14.1 5.71,14.86 v5.71,15.88 4.19,14.35 4.19,4.7 5.97,2.92 8.89,2.92 | v8.76,3.05 8.89,2.92 | 8.89,2.92 10.16,1.65 26.8,1.65 29.59,4.44 | v29.72,5.08 29.72,4.57 29.59,4.44 | v14.86,18.41 13.08,18.41 12.19,17.53 | v33.19,5.71 31.91,4.44 29.59,4.44
  pour Bottom: 1.14,63.12 67.94,63.12 68.07,62.99 68.07,0.51 0.89,0.51 0.89,63.25 1.14,63.25
5V_IN
  Top 0.203: J3.2 9.02,58.8 | J1.1 5.3,29.62 5.33,29.59 5.97,30.23 5.97,33.15 5.59,33.53 1.4,33.53 1.14,33.78 1.14,58.55 2.29,59.69 8.13,59.69 9.02,58.8 | U$1.2 28.12,62.24 23.65,62.24 23.25,61.85 10.92,61.85 9.02,59.94 9.02,58.8
CS_LLS  (1 unrouted)
DI_LLS  (1 unrouted)
GND  (via drill 0.35)  (2 unrouted)
  Top 0.203: J1.5 4.86,27.05 v6.22,27.05 | v10.03,4.44 J2.5 J2.7 v11.3,4.32 | U1.20 23.86,29.61 22.48,29.61 21.97,30.12 | U1.19 23.87,30.12 21.97,30.12 | 21.97,30.12 C15.2 19.05,31.51 v19.05,31.62 20.36,31.62 C1.1 | U1.99 26.25,43.89 C6.2 v27.43,43.94 28.75,43.94 R3.2 28.83,46.99 | C12.2 38.14,21.97 37.85,21.97 | 37.85,21.97 C8.2 34.81,23.37 v33.91,23.37 33.66,23.37 33.27,22.99 33.27,20.32 33.02,20.07 32.33,20.07 D2.C 32.26,18.41 31.24,17.4 | U1.74 41.57,38.65 42.67,39.75 42.67,40.51 42.15,41.04 C9.2 42.02,41.04 39.73,43.32 | C10.2 39.73,43.32 | 39.73,43.32 v38.61,44.45 36.72,44.45 C11.2 | C14.C 23.07,21 23.11,20.95 v23.05,20.89 | C16.C 13.97,29.34 | 13.97,29.34 v13.97,27.56 | D1.C 30.23,18.41 31.24,17.4 | 31.24,17.4 v31.24,16.26 | C18.2 v11.56,39.24 11.56,40.13 | C17.2 21.07,50.31 21.84,49.53 | 21.84,49.53 v22.86,49.53 26.29,49.53 28.83,46.99 | 21.84,49.53 21.72,49.53 21.23,49.04 C20.2 C19.2 21.23,42.56 19.94,41.28 v19.81,41.28 20.81,41.28 C7.2 | S1.3 9.83,38.4 11.56,40.13 | 11.56,40.13 11.56,42.24 9.88,43.92 | U2.2 U2.7 31.24,8.13 v31.24,10.03 | 28.83,46.99 29.34,47.5 v29.34,48.51 | U1.10 21.74,34.65 20.83,35.56 v20.45,35.56 | U1.49 37.25,23.07 37.85,22.48 37.85,21.97 | J2.11 13.84,5.46 13.72,5.33 v13.72,4.44 | C3.2 9.4,15.88 10.16,16.64 10.16,18.41 9.78,18.8 C5.2 9.16,20.19 10.69,21.72 12.41,21.72 C4.2 C2.2 v14.86,23.88 | J3.1 6.48,56.77 5.33,55.63 4.57,55.63 | 4.57,55.63 3.3,55.63 v3.17,55.5 | v6.1,48.64 6.1,47.13 C21.2 7.49,47.12 9.88,44.73 9.88,43.92 | D3.C 5.26,54.93 4.57,55.63 | J3.14 J3.13 v36.96,55.37 | v26.92,21.97 26.16,22.73 26.16,23.38 26.25,23.46 U1.27 | S1.4 7.71,44.45 9.35,44.45 9.88,43.92
  Top 0.203: 13.97,29.34 14.88,30.24 C13.2 17.27,30.86 16.89,31.24 v16.76,31.24
  pour Route2: 0.76,63.12 68.07,63.12 68.07,0.51 0.76,0.51
MISO  (1 unrouted)
MOSI  (1 unrouted)
N$1
  Top 0.203: R2.1 32.25,23.3 U1.39
N$2
  Top 0.203: R1.1 30.23,24 30.48,24.26 31.11,24.26 31.25,24.39 U1.37
N$3
  Top 0.203: D1.A R1.2
N$4
  Top 0.203: D2.A R2.2
N$5
  Top 0.203: U1.94 28.75,42.92 R3.1
N$6
  Top 0.203: U1.93 29.25,42.46 29.59,42.8 29.59,45.21 30.28,45.9 R4.1
N$7
  Top 0.203: U1.92 29.75,42.32 30.43,43 R5.1
N$8
  Top 0.203: D3.A 7.24,54.1 7.49,53.85 7.49,53.34 7.11,52.96 5.97,52.96 5.28,52.27 R6.1
N$10
  Top 0.203: C1.2 22.48,31.71 22.48,30.86 22.69,30.65 U1.18
N$12
  Top 0.203: C18.1 11.56,36.45 | 11.56,36.45 11.56,35.43 12.19,34.8 15.24,34.8 15.88,34.16 R8.2 | 11.56,36.45 12.06,35.94 13.39,35.94 Y1.1
N$13  (1 unrouted)
N$15  (1 unrouted)
N$17  (1 unrouted)
N$21  (1 unrouted)
NRST
  Top 0.203: U1.14 21.71,32.65 21.21,33.15 16.26,33.15 14.99,34.42 9.53,34.42 | S1.1 3.43,38.62 3.43,35.43 | 9.53,34.42 4.45,34.42 3.43,35.43 | 3.43,35.43 2.54,36.32 1.91,36.32 1.52,36.7 1.52,44.28 1.65,44.4 S1.2 3.43,44.62 3.43,46.23 | 3.43,46.23 4.32,47.12 C21.1 | 3.43,46.23 3.43,49.4 4.06,50.04 R9.1 5.33,50.09 5.33,50.8 5.59,51.05 10.16,51.05 J3.5 | J2.12 13.84,8.76 14.48,8.13 14.48,2.39 13.34,1.25 2.44,1.25 1.91,1.78 1.91,21.84 2.79,22.73 4.83,22.73 7.62,25.53 7.62,32.51 9.53,34.42
PC14-OSC32-IN
  Top 0.203: U1.8 22.77,35.65 21.84,36.58 21.84,37.91 Y2.2 21.91,39.56 21.34,40.13 19.05,40.13 18.8,40.39 18.8,43.31 19.3,43.82 C19.1
PC15-OSC32-OUT
  Top 0.203: U1.9 22.13,35.15 20.51,36.77 Y2.1 20.51,38.42 20.45,38.48 20.45,38.99 19.81,39.62 18.67,39.62 18.29,40.01 18.29,45.59 19.05,46.36 C20.1
PH0-OSC-IN
  Top 0.203: U1.12 21.85,33.65 20.83,34.67 19.68,34.67 16.89,37.47 16.89,43.31 | C17.1 18.92,49.15 18.16,48.39 17.27,48.39 16.89,48.01 16.89,43.31 | 16.89,43.31 16.26,43.94 15.88,43.94 15.49,44.32 Y1.2
PH1-OSC-OUT
  Top 0.203: U1.13 21.72,33.15 20.7,34.16 R8.1
SCK  (1 unrouted)
SCK_LLS  (1 unrouted)
SWCLK
  Top 0.203: J2.9 12.57,3.94 11.68,3.05 10.16,3.05 9.4,3.81 9.4,8.13 9.02,8.51 8.76,8.51 8.13,9.14 8.13,12.32 8.26,12.45 9.91,12.45 10.03,12.32 J2.6 10.03,8.74 10.16,8.61 11.4,8.61 11.94,9.14 11.94,15.11 12.57,15.75 22.86,15.75 24.26,17.14 24.26,24.77 25.35,25.85 25.35,26 26.01,26.67 32.38,26.67 37.75,32.04 U1.76
SWDIO
  Top 0.203: U1.72 41.35,37.65 42.8,36.2 42.93,36.07 43.18,35.81 43.18,18.03 40.39,15.24 15.11,15.24 14.73,14.86 14.48,14.61 13.21,13.34 13.21,9.14 12.32,8.26 9.78,8.26 8.76,9.27 J2.4
SWO
  Top 0.203: U1.89 31.25,38.62 25.02,32.39 25.02,27.05 24.64,26.67 21.84,26.67 21.47,26.3 21.47,22.11 21.32,21.96 17.77,21.96 14.86,24.86 14.86,24.89 7.75,24.89 3.94,21.08 3.94,15.49 4.7,14.73 10.54,14.73 11.3,13.96 J2.8
USART_RX  (via drill 0.35)
  Top 0.203: U1.87 32.25,43.17 32.89,43.81 v32.89,48.38 v32.89,48.39 31.88,49.4 J3.11 | v46.86,48.26 46.86,5.59 44.45,3.17 16.26,3.17 15.11,4.32 J2.13
  Bottom 0.203: v32.89,48.39 46.74,48.39 v46.86,48.26
USART_TX
  Top 0.203: U1.86 32.75,42.28 34.42,43.94 34.42,54.48 | J3.12 34.42,54.48 | 34.42,54.48 45.59,43.31 45.59,16 42.93,13.34 17.78,13.34 J2.14
VDDA
  Top 0.203: FB1.1 19.94,26.42 | 19.94,26.42 20.57,26.42 21.59,27.43 21.59,28.19 22.04,28.65 U1.22 | FB1.1 17.27,28.74 C13.1 | FB1.1 19.6,27.22 20.37,27.99 R7.2 | C14.A 19.94,23.29 19.94,26.42
VREF_PLUS
  Top 0.203: U1.21 23.82,29.07 C15.1 20.07,29.07 | 20.07,29.07 19.96,29.07 16.81,32.21 C16.A | R7.1 19.51,28.51 20.07,29.07

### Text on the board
tPlace: Alexander Robles

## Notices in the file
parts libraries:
SparkFun-Connectors: Licensing: Creative Commons ShareAlike 4.0 International - https://creativecommons.org/licenses/by-sa/4.0
